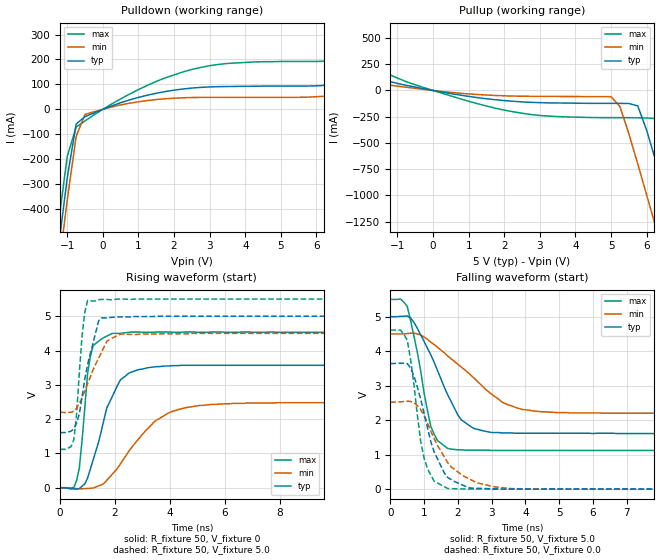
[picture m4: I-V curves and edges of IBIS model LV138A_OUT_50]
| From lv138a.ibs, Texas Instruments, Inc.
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|   Model LV138A_OUT_50
[Model]   LV138A_OUT_50
Model_type  Output
Polarity   Non-Inverting
Vmeas = 2.50v
Cref = 15pf
| variable   typ   min   max
C_comp   4.62pf   3.47pf   5.77pf
[Temperature Range]   25   85   -40
[Voltage Range]   5.0   4.5   5.5
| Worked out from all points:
|   slope of the pulldown table from 0 to 0.75 V, typ, clamps not added: 19.9 ohm
|   slope of the pullup table from 0 to 0.75 V, typ, clamps not added: 17.2 ohm
|   rising waveform, R_fixture 50, V_fixture 0: 20-80 % time 851ps typ, 1.53ns min, 320ps max; typ from 0 V to 3.57 V
|   falling waveform, R_fixture 50, V_fixture 5.0: 20-80 % time 949ps typ, 1.64ns min, 502ps max; typ from 5 V to 1.61 V
|   rising waveform, R_fixture 50, V_fixture 5.0: 20-80 % time 506ps typ, 747ps min, 247ps max; typ from 1.61 V to 5 V
|   falling waveform, R_fixture 50, V_fixture 0.0: 20-80 % time 657ps typ, 939ps min, 385ps max; typ from 3.64 V to 0 V
[Pulldown]
|   Voltage   I(typ)   I(min)   I(max)
-5V       -5.14A     -5.22A     -5.05A
-1.5V     -853mA     -945mA     -756mA
-1.25V    -557mA     -649mA     -461mA
-1V       -274mA     -363mA     -188mA
-750mV    -58.9mA    -108mA     -71.3mA
-500mV    -29.2mA    -20mA      -46.2mA
0V        -3.33nA    -3.4nA     -3.57nA
1.25V     56.7mA     35.2mA     96mA
2.5V      85.3mA     47.3mA     160mA
3.5V      91.4mA     47.8mA     184mA
6.75V     103mA      58.5mA     199mA
10V       179mA      107mA      329mA
[Pullup]
|   Voltage   I(typ)   I(min)   I(max)
-5V       317mA      173mA      595mA
-3.5V     253mA      144mA      466mA
-750mV    48.6mA     30.8mA     83.5mA
1.5V      -78.8mA    -43.4mA    -148mA
5V        -123mA     -58.9mA    -259mA
5.25V     -123mA     -153mA     -259mA
5.75V     -147mA     -699mA     -260mA
6.25V     -664mA     -1.29A     -268mA
6.5V      -960mA     -1.6A      -403mA
6.75V     -1.26A     -1.9A      -685mA
7.25V     -1.87A     -2.51A     -1.28A
10V       -5.25A     -5.89A     -4.66A
[Ramp]
| variable   typ   min   max
dV/dt_r   2.15E+00/7.55E-10   1.50E+00/1.55E-09   2.72E+00/3.02E-10
dV/dt_f   2.05E+00/9.47E-10   1.39E+00/1.63E-09   2.64E+00/5.48E-10
R_load = 50
[Rising Waveform]
R_fixture = 50
V_fixture = 0
|   Time   V(typ)   V(min)   V(max)
0s        0V         0V         0V
600ps     -40.3mV    -24mV      210mV
700ps     -21.6mV    -26.7mV    581mV
1ns       283mV      -19.2mV    3.33V
1.2ns     806mV      -8.42mV    4.14V
1.9ns     2.66V      397mV      4.5V
2.5ns     3.34V      1.06V      4.53V
3.5ns     3.53V      1.97V      4.54V
5.1ns     3.57V      2.4V       4.53V
25ns      3.57V      2.48V      4.53V
[Falling Waveform]
R_fixture = 50
V_fixture = 5.0
V_fixture_min = 4.5
V_fixture_max = 5.5
|   Time   V(typ)   V(min)   V(max)
0s        5V         4.5V       5.5V
500ps     5.02V      4.51V      5.3V
1.2ns     3.89V      4.26V      1.81V
1.4ns     3.43V      4.11V      1.4V
1.8ns     2.54V      3.78V      1.16V
2.1ns     2.01V      3.54V      1.14V
2.5ns     1.75V      3.2V       1.13V
3.4ns     1.63V      2.48V      1.12V
4.5ns     1.62V      2.24V      1.12V
25ns      1.61V      2.2V       1.12V
[Rising Waveform]
R_fixture = 50
V_fixture = 5.0
V_fixture_min = 4.5
V_fixture_max = 5.5
|   Time   V(typ)   V(min)   V(max)
0s        1.61V      2.2V       1.12V
500ps     1.72V      2.23V      1.41V
600ps     1.88V      2.32V      2.15V
800ps     2.66V      2.63V      4.45V
900ps     3.18V      2.82V      5.12V
1ns       3.59V      3.03V      5.46V
1.4ns     4.86V      3.77V      5.48V
1.7ns     4.95V      4.27V      5.49V
2.2ns     4.98V      4.48V      5.5V
25ns      5V         4.5V       5.5V
[Falling Waveform]
R_fixture = 50
V_fixture = 0.0
|   Time   V(typ)   V(min)   V(max)
0s        3.64V      2.52V      4.61V
500ps     3.64V      2.55V      4.32V
700ps     3.28V      2.51V      3.02V
900ps     2.6V       2.3V       1.38V
1ns       2.19V      2.13V      898mV
1.3ns     1.07V      1.46V      228mV
1.7ns     337mV      765mV      18.2mV
2.5ns     25.8mV     213mV      2.95mV
3.6ns     1.93mV     14.9mV     1.31mV
25ns      9.43uV     2.74uV     8.26uV
